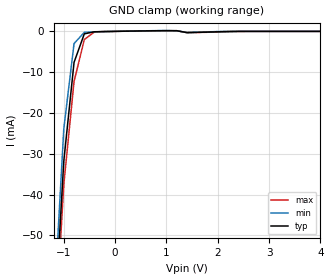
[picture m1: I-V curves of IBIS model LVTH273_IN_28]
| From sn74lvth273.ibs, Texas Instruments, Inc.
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|   Model LVTH273_IN_28
[Model]   LVTH273_IN_28
Model_type  Input
Polarity   Non-Inverting
Vinl = 0.8
Vinh = 2.0
| variable   typ   min   max
C_comp   4pf   NA   NA
[Temperature Range]   40   -25   100
| Ambient temperature   25   -40   85
[Voltage range]   2.8   2.7   2.9
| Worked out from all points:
|   GND clamp passes 1 mA (typ) near -0.61 V on its own axis
[GND Clamp]
|   Voltage   I(typ)   I(min)   I(max)
-5V       -1.687A    -1.924A    -1.502A
-1.2V     -75.69mA   -69.7mA    -80.63mA
-1V       -31.82mA   -23.89mA   -37.56mA
-800mV    -7.59mA    -2.979mA   -12.25mA
-600mV    -601.9uA   -239.6uA   -2.007mA
-400mV    -97.79uA   -110.2uA   -123.1uA
-200mV    -46.79uA   -53.84uA   -41.55uA
1.2V      166uA      136.7uA    161uA
1.4V      -300.4uA   -269.7uA   -320.6uA
2.4V      -654.8nA   -343.4pA   -28.73uA
5V        -619.8pA   309.3pA    633.9pA
